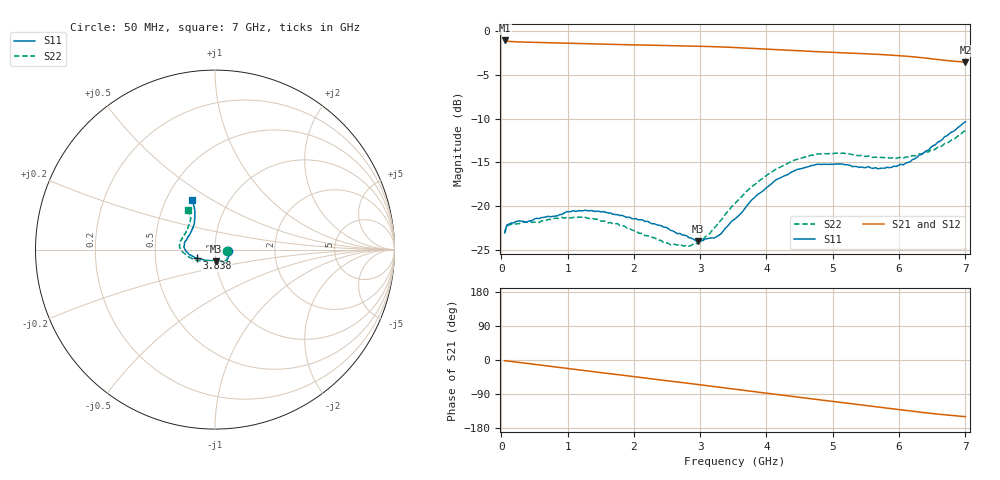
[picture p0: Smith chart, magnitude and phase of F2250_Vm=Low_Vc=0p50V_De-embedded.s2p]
! Integrated Device Technology
! Corporate Headquarters
! 6024 Silver Creek Valley Road
! San Jose, CA 95138  USA
! Phone:  1-408-284-8200
! Toll Free:  1-800-223-1366
! Webpage:  http://www.idt.com/
! Timing and RF Division
! 515 Groton Road, Suite 102
! Westford, MA 01886-6024
! Device:  F2250
! Description: Voltage Variable RF Attenuator
! Frequency:  50.0 -  6000.00 MHz
! Package:  3x3 mm Thin QFN Plastic Package: 16 pin
! Ports:  2 RF, 3 DC
!  Pin  1  = GND
!  Pin  2  = NC
!  Pin  3  = RF1  = Port 1
!  Pin  4  = NC
!  Pin  5  = GND
!  Pin  6  = GND
!  Pin  7  = GND
!  Pin  8  = GND
!  Pin  9  = NC
!  Pin 10  = RF2  = Port 2
!  Pin 11  = NC
!  Pin 12  = GND
!  Pin 13  = GND
!  Pin 14  = VCNTRL
!  Pin 15  = VDD
!  Pin 16  = VMODE
! Vcntrl:  0.500 Volts
! Vmode:  +0.000 Volts
! Vdd:  +3.30  Volts
! Current:  1.132 mA
! Data:  The device was measured on a the F2250 evaluation board which has
!  individual transmission lines to the RF pins.  Data was collected
!  using a calibrated network analyzer.  The evaluation board was
!  de-embedded using a TRL calibration technique.
!  The reference plane is the edge of the package pin.
! Misc:  SN 10
!  Action Tracker AT0258
! Date Measured:  2014-11-26
! Date:  2015-10-15  MJV
! Note:
!  Integrated Device Technology supplies this data as a sample of measured
!  data at the package pin for this product.  Your particular data for this
!  product may vary.
!  Data was taken at 25 degrees C.
!  Integrated Device Technology reserves the right to change this data at anytime.
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# GHz S dB R 50
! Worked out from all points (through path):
!   201 points, 50 MHz to 7 GHz, reference 50 ohm
!   highest |S21| = -1.08 dB at 50 MHz (marker M1); lowest = -3.6 dB at 7 GHz (marker M2)
!   group delay of S21, straight-line fit = 60.1 ps
!   lowest |S11| = -24.0 dB at 2.969 GHz (marker M3), VSWR 1.13, Z = 50.2 - j6.34 ohm
!   |S11| at or under -10 dB: start of sweep to end of sweep
!   |S22| runs from -24.6 to -11.4 dB; largest |S21 - S12| = 0.00039
!   S11 on the Smith chart (normalised r, x): 50 MHz: 1.15, -0.02; 3.838 GHz: 0.81, -0.08; 7 GHz: 0.67, +0.41
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0.05  -22.95 -7.7  -1.08 -1.8  -1.08 -1.8  -23.15 -8.6
0.08475  -22.17 -7.7  -1.16 -2.5  -1.16 -2.5  -22.30 -8.1
0.15425  -21.94 -9.8  -1.21 -4.0  -1.21 -4.0  -22.07 -9.8
0.71025  -21.17 -33.0  -1.34 -16.2  -1.34 -16.2  -21.51 -35.5
1.2315  -20.55 -49.5  -1.46 -27.4  -1.45 -27.4  -21.33 -55.8
1.75275  -20.99 -56.3  -1.55 -38.5  -1.55 -38.5  -21.99 -64.4
2.37825  -22.20 -58.1  -1.64 -51.8  -1.64 -51.8  -23.88 -70.3
2.552  -22.78 -61.6  -1.66 -55.6  -1.66 -55.6  -24.43 -76.1
2.7605  -23.34 -70.2  -1.70 -60.2  -1.70 -60.2  -24.58 -87.4
2.969  -23.99 -84.3  -1.74 -64.8  -1.73 -64.8  -24.12 -103.1
3.247  -23.50 -111.6  -1.80 -71.0  -1.80 -71.0  -22.22 -125.9
3.525  -21.48 -137.0  -1.89 -77.2  -1.89 -77.2  -19.71 -143.0
3.83775  -18.89 -155.1  -2.00 -84.1  -2.00 -84.1  -17.46 -157.1
4.1505  -16.97 -167.6  -2.13 -90.9  -2.13 -90.9  -15.77 -169.2
4.4285  -15.94 -175.8  -2.23 -97.0  -2.23 -97.0  -14.73 -176.7
4.7065  -15.34 177.1  -2.34 -103.0  -2.34 -103.0  -14.19 177.1
5.15825  -15.22 166.2  -2.50 -112.7  -2.50 -112.7  -13.95 167.6
5.85325  -15.61 142.5  -2.74 -127.6  -2.75 -127.7  -14.53 152.1
6.166  -14.94 131.0  -2.91 -134.4  -2.91 -134.5  -14.38 143.1
6.444  -13.60 122.0  -3.12 -140.2  -3.12 -140.3  -13.81 133.7
6.82625  -11.45 115.8  -3.44 -146.9  -3.44 -146.9  -12.38 125.6
7  -10.38 114.9  -3.56 -149.5  -3.56 -149.6  -11.38 124.1
